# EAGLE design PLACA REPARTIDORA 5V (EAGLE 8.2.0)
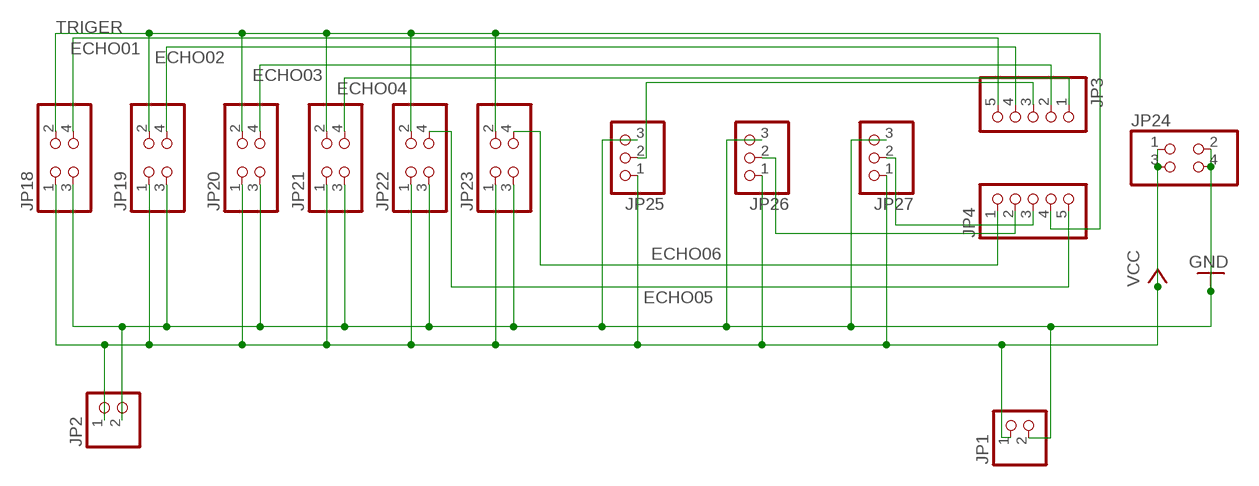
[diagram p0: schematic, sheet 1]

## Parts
JP1  PINHD-1X2  [1X02]
JP2  PINHD-1X2  [1X02]
JP3  PINHD-1X5  [1X05]
JP4  PINHD-1X5  [1X05]
JP18  PINHD-2X2  [2X02]
JP19  PINHD-2X2  [2X02]
JP20  PINHD-2X2  [2X02]
JP21  PINHD-2X2  [2X02]
JP22  PINHD-2X2  [2X02]
JP23  PINHD-2X2  [2X02]
JP24  PINHD-2X2  [2X02]
JP25  PINHD-1X3  [1X03]
JP26  PINHD-1X3  [1X03]
JP27  PINHD-1X3  [1X03]

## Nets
ECHO01: JP3.5 JP18.4
ECHO02: JP3.4 JP19.4
ECHO03: JP3.2 JP20.4
ECHO04: JP3.1 JP21.4
ECHO05: JP4.5 JP22.4
ECHO06: JP4.1 JP23.4
GND: JP1.2 JP2.2 JP18.3 JP19.3 JP20.3 JP21.3 JP22.3 JP23.3 JP24.2 JP24.4 JP25.3 JP26.3 JP27.3
N$6: JP3.3 JP25.2
N$10: JP4.2 JP26.2
N$11: JP4.3 JP27.2
TRIGER: JP4.4 JP18.2 JP19.2 JP20.2 JP21.2 JP22.2 JP23.2
VCC: JP1.1 JP2.1 JP18.1 JP19.1 JP20.1 JP21.1 JP22.1 JP23.1 JP24.1 JP24.3 JP25.1 JP26.1 JP27.1

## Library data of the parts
JP1 JP2 = pinhead:PINHD-1X2: PIN HEADER
JP3 JP4 = pinhead:PINHD-1X5: PIN HEADER
JP18-JP24 = pinhead:PINHD-2X2: PIN HEADER
JP25-JP27 = pinhead:PINHD-1X3: PIN HEADER

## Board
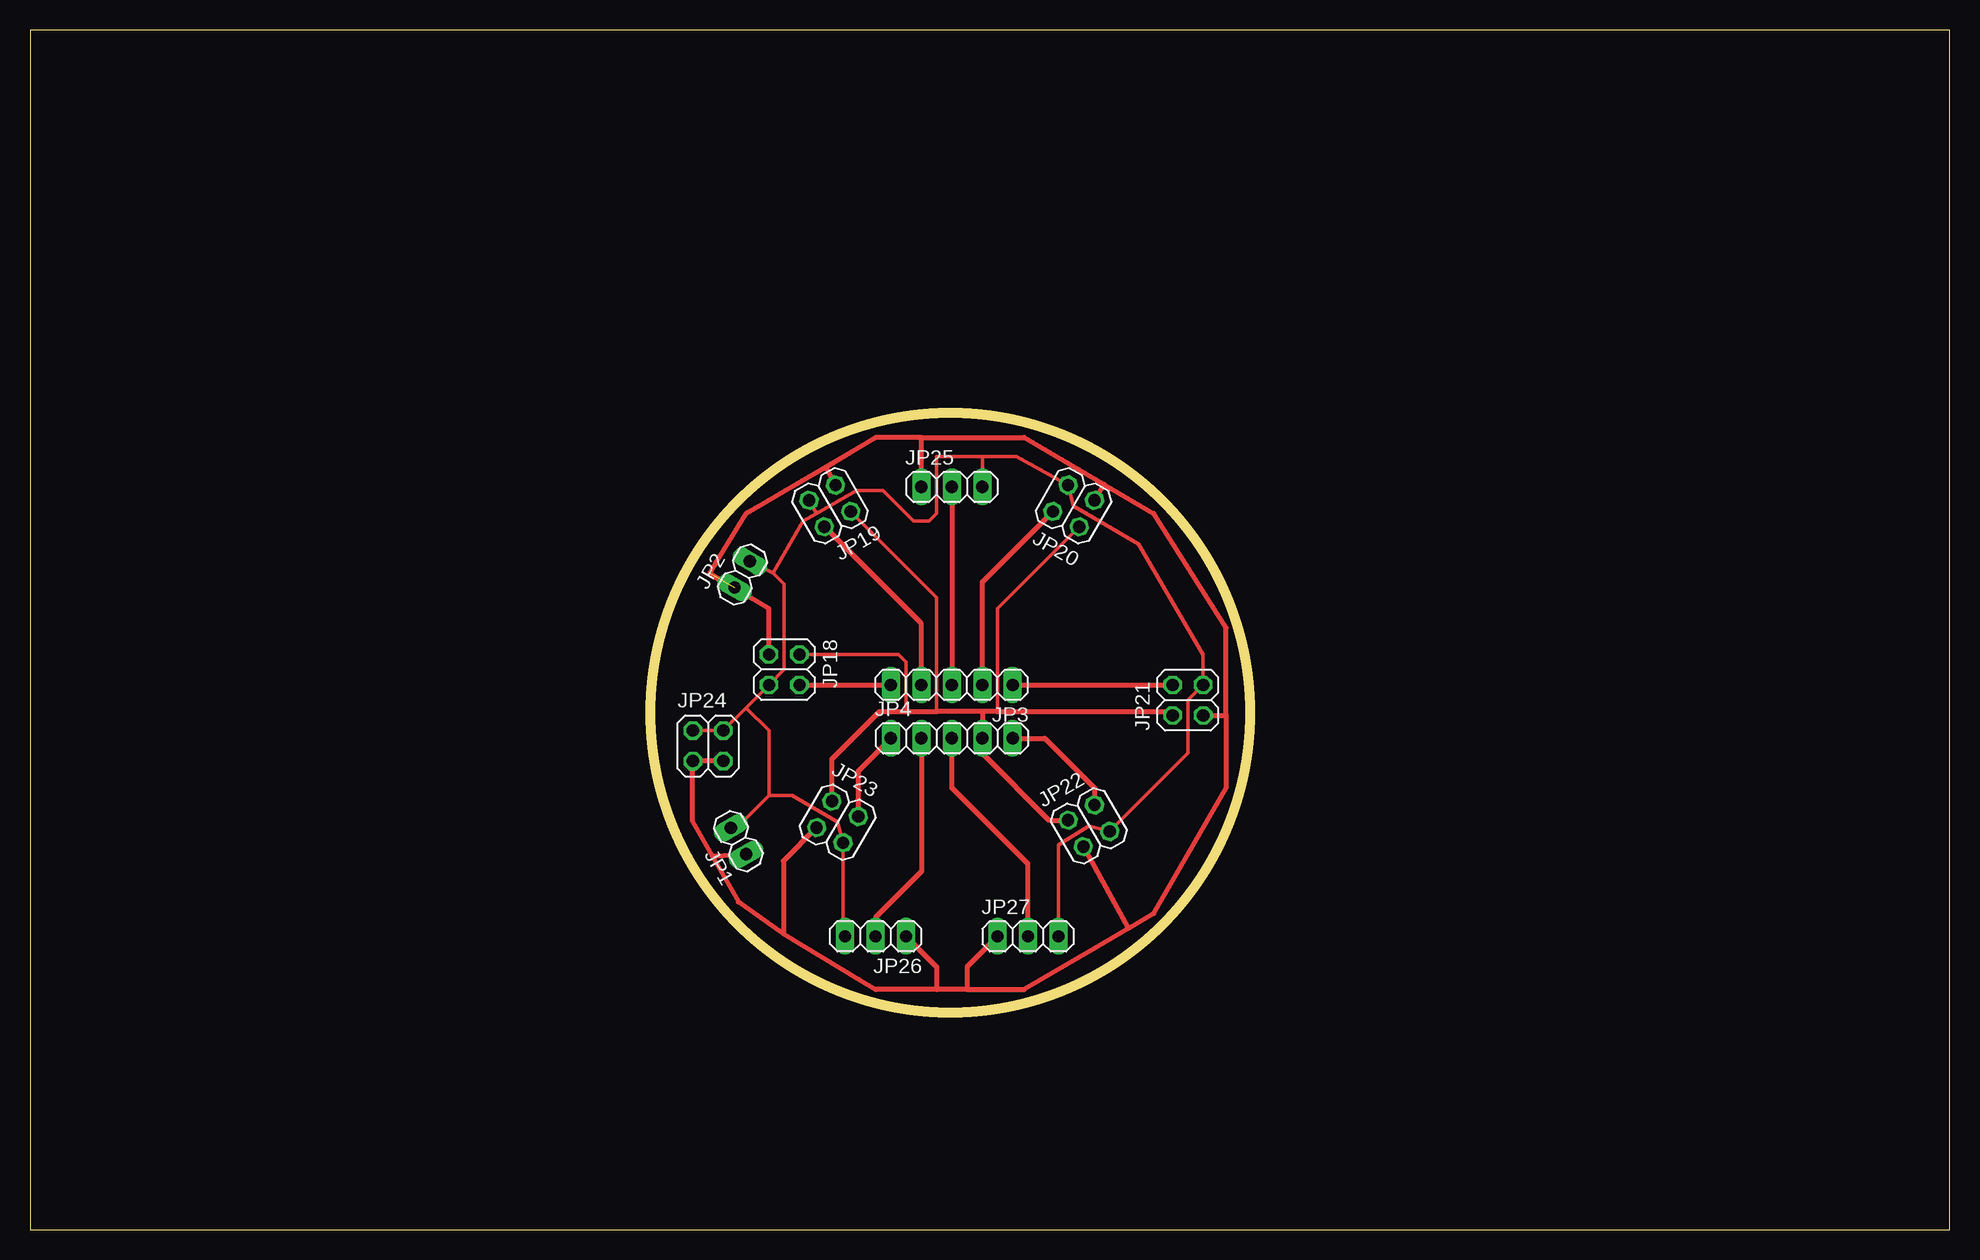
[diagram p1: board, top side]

Size 160 x 100 mm. Coordinates in mm from the lower left corner, seen from the top.
Outline: 0,0 160,0 160,100 0,100 0,0
Outline: circle at 76.71,43.08 radius 25
Copper layers (1*16): Top 0.035mm / dielectric 1.5mm / Bottom 0.035mm
Design rules "default": minimum track width 6mil, minimum drill 0.35mm, track to track 6mil, track to pad 6mil, pad to pad 6mil, via to via 6mil, smd to smd 6mil, copper to edge 40mil, drill to drill 6mil, minimum pad ring 10mil, minimum via ring 8mil, stop-mask expansion 4mil, vias tented up to drill 0mil, thermal gap 10mil

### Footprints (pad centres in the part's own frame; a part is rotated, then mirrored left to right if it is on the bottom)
1X02 = drill 1.016 long: 1 -1.27,0; 2 1.27,0
1X05 = drill 1.016 long: 1 -5.08,0; 2 -2.54,0; 3 0,0; 4 2.54,0; 5 5.08,0
2X02 = drill 1.016 octagon: 1 -1.27,-1.27; 2 -1.27,1.27; 3 1.27,-1.27; 4 1.27,1.27
1X03 = drill 1.016 long: 1 -2.54,0; 2 0,0; 3 2.54,0

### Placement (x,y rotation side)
JP1  59.05,32.38 120 top
JP2  59.37,54.61 60 top
JP3  76.83,45.4 180 top
JP4  76.83,40.96 0 top
JP18  62.87,46.67 270 top
JP19  66.67,60.33 210 top
JP20  87,60.33 150 top
JP21  96.52,44.13 90 top
JP22  88.27,33.66 30 top
JP23  67.31,33.97 330 top
JP24  56.52,40.32 0 top
JP25  76.83,61.91 0 top
JP26  70.48,24.45 180 top
JP27  83.19,24.45 0 top

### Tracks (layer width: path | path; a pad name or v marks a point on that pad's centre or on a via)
ECHO01
  Top 0.406: JP18.4 JP3.5
ECHO02
  Top 0.406: JP3.4 74.3,50.51 JP19.4
ECHO03
  Top 0.406: JP3.2 79.38,53.98 JP20.4
ECHO04
  Top 0.406: JP3.1 JP21.4
ECHO05
  Top 0.406: JP22.4 88.73,36.83 84.6,40.96 JP4.5
ECHO06
  Top 0.406: JP23.4 69.05,38.25 JP4.1
GND
  Top 0.305: JP19.3 65.54,59.7 | 79.38,64.45 82.23,64.45 JP20.3 87,60.33 92.39,57.15 97.79,47.94 JP21.3 96.52,44.13 96.52,39.71 JP22.3 88.27,33.66 85.72,32.07 JP27.3 | 79.38,64.45 75.56,64.45 75.56,59.69 74.93,59.05 73.66,59.05 71.12,61.59 68.9,61.59 65.54,59.7 | JP25.3 79.38,64.45 | 65.54,59.7 64.45,59.06 61.95,54.72 | JP2.2 61.95,54.72 | JP24.2 JP24.4 59.69,43.5 | 59.69,43.5 JP18.3 62.87,46.67 62.87,53.81 61.95,54.72 | 61.59,36.2 63.5,36.2 67.31,33.97 JP23.3 67.78,24.62 JP26.3 | 61.59,36.2 58.88,33.48 JP1.2 | 61.59,36.2 61.59,41.59 59.69,43.5
N$6
  Top 0.406: JP25.2 JP3.3
N$10
  Top 0.406: JP4.2 74.3,29.84 70.48,26.04 JP26.2
N$11
  Top 0.406: JP4.3 76.83,36.83 83.19,30.48 JP27.2
TRIGER
  Top 0.305: 75.56,43.18 75.56,52.7 JP19.2 | 80.64,43.18 80.64,51.77 JP20.2 | 73.03,43.18 73.03,47.31 72.39,47.94 JP18.2 | 85.09,34.12 84.94,34.12 79.38,39.69
  Top 0.406: 79.38,43.18 80.64,43.18 94.61,43.18 JP21.2 | 79.38,43.18 75.56,43.18 73.03,43.18 70.8,43.18 66.84,39.22 JP23.2 | 79.38,43.18 79.38,39.69 | JP4.4 79.38,39.69 | 79.38,39.69 84.94,34.12 | 85.09,34.12 JP22.2
VCC  (1 unrouted)
  Top 0.406: 70.48,66.04 66.34,63.53 | 74.3,66.04 70.48,66.04 | 74.3,66.04 82.87,66.04 89.53,62.12 | 89.53,62.12 93.66,59.69 99.69,50.16 99.69,42.86 | 99.69,42.86 99.69,36.83 93.66,26.35 91.55,25.11 | 91.55,25.11 88.74,23.45 82.87,20 78.11,20 | 78.11,20 75.56,20 | 75.56,20 70.48,20 69.13,20.82 62.8,24.66 | 62.8,24.66 59.05,27.3 56.85,31.13 | 56.85,31.13 55.19,34.08 55.19,39.05 JP24.1 JP24.3 | JP19.1 66.34,63.53 | JP25.1 74.3,66.04 | JP20.1 89.53,62.12 | JP21.1 99.69,42.86 | 56.85,31.13 JP1.1 | 66.34,63.53 59.69,59.69 | 59.69,59.69 57.12,55.46 57.03,55.32 56.61,54.62 61.59,51.75 | 59.69,59.69 70.48,66.04 | JP26.1 75.56,21.91 75.56,20 | JP27.1 78.11,21.91 78.11,20 | JP23.1 62.8,30.73 62.8,24.66 | JP22.1 91.55,25.11 | JP18.1 61.59,51.75 | 56.66,54.71 61.59,51.75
